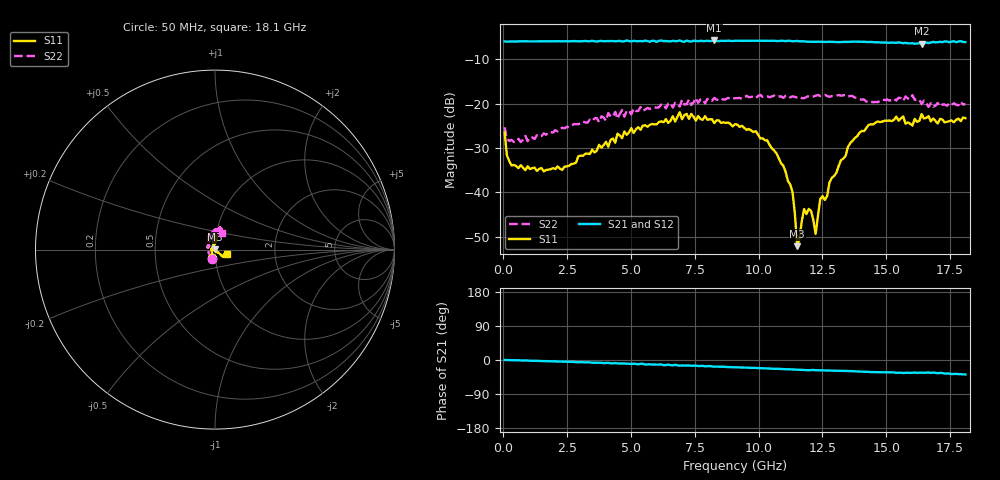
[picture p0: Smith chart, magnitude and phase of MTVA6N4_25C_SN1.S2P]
! Network Analyzer HP8720D.06.14 Serial No. US36140669
!  6 Jul 2005  07:09:45
! Frequency  S11  S21  S12  S22
# HZ  S  DB R 50
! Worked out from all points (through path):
!   201 points, 50 MHz to 18.1 GHz, reference 50 ohm
!   highest |S21| = -5.76 dB at 8.263 GHz (marker M1); lowest = -6.5 dB at 16.39 GHz (marker M2)
!   group delay of S21, straight-line fit = 6 ps
!   lowest |S11| = -52.1 dB at 11.51 GHz (marker M3), VSWR 1.00, Z = 49.8 + j0.192 ohm
!   |S11| at or under -10 dB: start of sweep to end of sweep
!   |S22| runs from -28.7 to -18.0 dB; largest |S21 - S12| = 0.016
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5e7  -26.48 -107.3  -5.97 0.1  -5.98 0.0  -25.33 -106.9
1.4025e8  -31.67 -131.4  -6.02 -0.1  -6.00 -0.1  -27.94 -151.1
3.2075e8  -33.94 -157.8  -5.97 -0.4  -5.99 -0.4  -28.19 -173.1
8.6225e8  -35.02 167.5  -5.97 -1.4  -5.97 -1.4  -27.26 166.3
3.1185e9  -31.76 111.3  -5.91 -5.9  -5.95 -6.2  -24.03 128.2
6.09675e9  -24.14 85.5  -5.84 -12.2  -5.75 -12.4  -20.83 99.9
6.909e9  -21.93 88.8  -5.76 -15.0  -5.86 -14.2  -20.64 89.3
8.26275e9  -24.39 91.8  -5.76 -17.5  -5.83 -18.1  -18.70 80.2
9.075e9  -24.65 94.3  -5.83 -19.1  -5.81 -19.1  -18.78 78.6
1.03385e10  -28.30 105.5  -5.83 -22.3  -5.84 -22.5  -18.36 72.6
1.097025e10  -34.05 112.1  -5.85 -23.9  -5.87 -24.2  -18.69 74.1
1.133125e10  -40.02 113.5  -5.94 -24.9  -5.90 -25.2  -18.35 75.0
1.151175e10  -52.14 128.8  -5.87 -25.3  -5.88 -25.7  -18.58 75.0
1.17825e10  -43.77 -119.7  -5.96 -26.3  -5.97 -26.8  -18.79 77.9
1.21435e10  -46.27 -97.1  -6.07 -26.4  -6.01 -26.7  -18.39 79.5
1.223375e10  -49.39 -98.3  -6.07 -26.9  -6.06 -27.1  -18.19 78.2
1.241425e10  -41.51 -87.1  -6.06 -27.2  -6.03 -27.3  -18.29 79.1
1.2685e10  -40.85 -63.8  -6.07 -27.6  -6.07 -27.6  -18.29 78.0
1.35875e10  -28.93 -40.6  -6.06 -29.1  -6.02 -29.4  -18.27 74.8
1.512175e10  -23.80 -36.6  -6.29 -32.9  -6.15 -32.9  -19.31 79.8
1.638525e10  -22.36 -21.3  -6.49 -33.1  -6.35 -33.2  -20.12 68.5
1.81e10  -23.27 -19.7  -6.12 -38.1  -6.22 -38.5  -20.07 67.0
